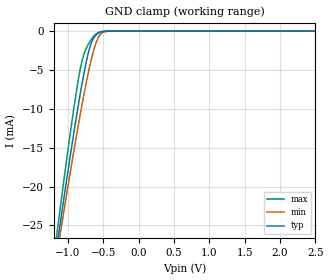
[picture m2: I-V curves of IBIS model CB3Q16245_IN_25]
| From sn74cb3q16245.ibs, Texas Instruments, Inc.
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[Model]   CB3Q16245_IN_25
Model_type  Input
Vinl=0.7
Vinh=1.7
| variable   typ   min   max
C_comp   2.28pF   1.80pF   2.84pF
[Temperature Range]   40   100   -40
| Ambient temperature   25   85   -40
[Voltage range]   2.5   2.3   2.7
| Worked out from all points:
|   GND clamp passes 1 mA (typ) near -0.64 V on its own axis
[GND Clamp]
| CB3Q16245_IN_25
|   Voltage   I(typ)   I(min)   I(max)
-5.5V     -337.1mA   -312.5mA   -365.5mA
-1.17V    -28.55mA   -29.6mA    -27.04mA
-1.13V    -26.02mA   -27.29mA   -24.21mA
-1.095V   -23.83mA   -25.29mA   -21.76mA
-925mV    -13.57mA   -15.86mA   -10.43mA
-825mV    -8.012mA   -10.65mA   -4.845mA
-775mV    -5.5mA     -8.197mA   -3.007mA
-700mV    -2.405mA   -4.831mA   -1.502mA
-590mV    -395.9uA   -1.206mA   -292.5uA
-515mV    -88.12uA   -229.6uA   -44.87uA
-395mV    -4.232uA   -9.382uA   -775nA
2.5V      57.25pA    176.5pA    32.61pA
